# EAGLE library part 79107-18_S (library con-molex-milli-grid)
RECEPTACAL
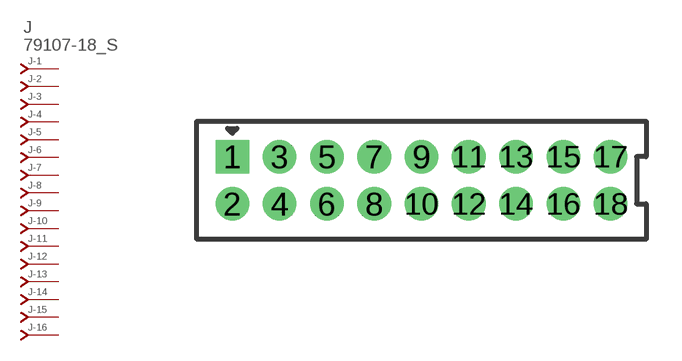
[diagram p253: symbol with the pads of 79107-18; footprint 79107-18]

Designator prefix J; gates -1=J-NV -2=J-N -3=J-N -4=J-N -5=J-N -6=J-N -7=J-N -8=J-N -9=J-N -10=J-N -11=J-N -12=J-N -13=J-N -14=J-N -15=J-N -16=J-N -17=J-N -18=J-N

## 79107-18_S  [79107-18]
1  -1:J  pas
2  -2:J  pas
3  -3:J  pas
4  -4:J  pas
5  -5:J  pas
6  -6:J  pas
7  -7:J  pas
8  -8:J  pas
9  -9:J  pas
10  -10:J  pas
11  -11:J  pas
12  -12:J  pas
13  -13:J  pas
14  -14:J  pas
15  -15:J  pas
16  -16:J  pas
17  -17:J  pas
18  -18:J  pas

## Footprint 79107-18 (pad centres in mm)
RECEPTACAL Dual Row, Vertical, Through-Hole
drill 0.914 square: 1 -8,1
drill 0.914: 2 -8,-1; 3 -6,1; 4 -6,-1; 5 -4,1; 6 -4,-1; 7 -2,1; 8 -2,-1; 9 0,1; 10 0,-1; 11 2,1; 12 2,-1; 13 4,1; 14 4,-1; 15 6,1; 16 6,-1; 17 8,1; 18 8,-1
